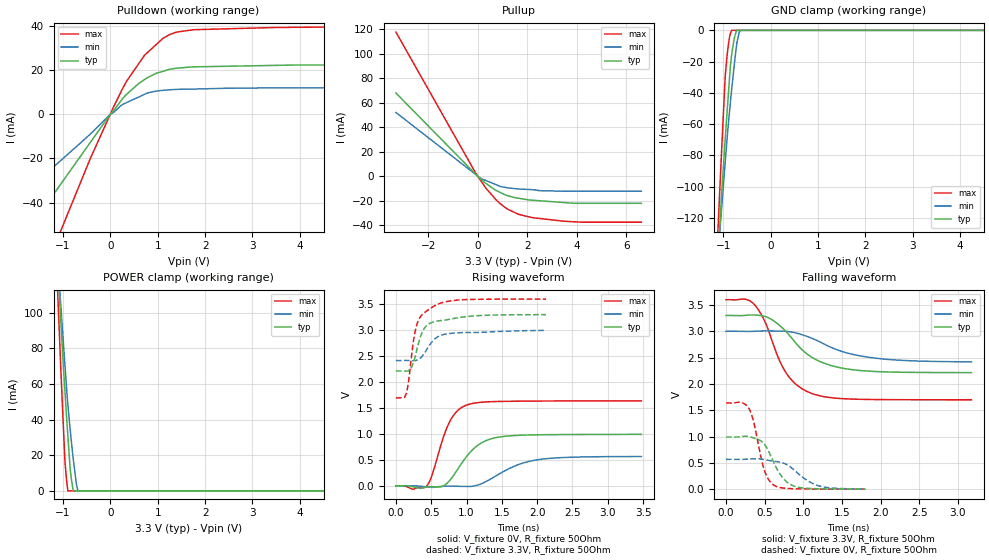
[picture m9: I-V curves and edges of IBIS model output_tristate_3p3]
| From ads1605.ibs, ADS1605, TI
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|   OUTPUT 3.3V Model
[Model]   output_tristate_3p3
Model_type   3-state
Polarity   Non-Inverting
Enable   Active-Low
Vmeas = 1.65
Vref = 1.65
Cref = 15pF
Rref = 50
|   typ   min   max
|   (nom PVT)   (Fast PVT)   (Slow PVT)
|Average
C_comp   2.296e-12   2.043e-12   2.570e-12
|ON state : BUFFER OUTPUT TURNED HIGH
|C_comp   2.372e-12   2.654e-12   2.116e-12
|OFF state: BUFFER in HIGH IMPEDANCE for IOs and 3-state
|C_comp   2.221e-12   2.485e-12   1.971e-12
|Where nom PVT is NOM Process, 3.3V,39C
|   Fast PVT is Strong Process, 3.6V, -40C
|   Slow PVT is Weak Process, 3.0V, 99C
[Voltage Range]   3.3   3   3.6
|Ambient Temperature   25   85   -40
|Junction Temperature
[Temperature Range]   39   99   -40
[Pullup Reference]   3.3   3   3.6
[Pulldown Reference]   0   0   0
[Power Clamp Reference]   3.3   3   3.6
[GND Clamp Reference]   0   0   0
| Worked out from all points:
|   slope of the pulldown table from 0 to 0.495 V, typ, clamps not added: 41.7 ohm
|   slope of the pullup table from 0 to 0.495 V, typ, clamps not added: 60.5 ohm
|   GND clamp passes 1 mA (typ) near -0.73 V on its own axis
|   POWER clamp passes 1 mA (typ) near -0.79 V on its own axis
|   falling waveform, V_fixture 3.3V, R_fixture 50Ohm: 20-80 % time 491ps typ, 647ps min, 355ps max; typ from 3.3 V to 2.21 V
|   rising waveform, V_fixture 0V, R_fixture 50Ohm: 20-80 % time 357ps typ, 516ps min, 253ps max; typ from 0 V to 0.991 V
|   rising waveform, V_fixture 3.3V, R_fixture 50Ohm: 20-80 % time 171ps typ, 211ps min, 144ps max; typ from 2.21 V to 3.3 V
|   falling waveform, V_fixture 0V, R_fixture 50Ohm: 20-80 % time 220ps typ, 309ps min, 152ps max; typ from 0.992 V to 0.002 V
[Pulldown]
|   Voltage   I(typ)   I(min)   I(max)
-3.3V     -99.75mA   -64.03mA   -170.9mA
-429mV    -12.97mA   -9.156mA   -20.36mA
0V        0A         0A         0A
346.8mV   9.051mA    5.259mA    15.01mA
721.2mV   15.6mA     8.938mA    26.62mA
957mV     18.37mA    10.36mA    31.26mA
1.11V     19.37mA    10.77mA    34.28mA
1.254V    20.3mA     11.01mA    35.99mA
1.434V    20.81mA    11.22mA    37.22mA
1.769V    21.38mA    11.33mA    38.18mA
3.45V     22.03mA    11.88mA    39.16mA
6.6V      22.2mA     11.88mA    39.35mA
[GND Clamp]
|   Voltage   I(typ)   I(min)   I(max)
-3.3V     -1.369A    -1.09A     -1.846A
-1.154V   -167.2mA   -161.9mA   -157.2mA
-1.086V   -131.4mA   -134.2mA   -110.6mA
-1.065V   -120.5mA   -125.8mA   -96.82mA
-956.4mV  -68.89mA   -83.51mA   -28.89mA
-877.2mV  -34.64mA   -55.08mA   -6.148mA
-848.1mV  -22.38mA   -45.89mA   -1.939mA
-819.6mV  -15.04mA   -37.07mA   0A
-765.6mV  -4.996mA   -21.71mA   0A
-714mV    -202uA     -8.333mA   0A
-643.5mV  0A         0A         0A
6.6V      0A         0A         0A
[Pullup]
|   Voltage   I(typ)   I(min)   I(max)
-3.3V     67.86mA    51.99mA    117.6mA
0V        0A         0A         0A
332.4mV   -5.843mA   -3.458mA   -9.787mA
764.4mV   -11.7mA    -7.032mA   -19.71mA
1.096V    -15.02mA   -8.994mA   -25.29mA
1.646V    -17.89mA   -10.35mA   -30.99mA
2.194V    -19.48mA   -10.9mA    -33.7mA
2.433V    -19.84mA   -11.69mA   -34.24mA
3.45V     -21.37mA   -12.17mA   -36.56mA
4.202V    -22.03mA   -12.17mA   -37.42mA
6.6V      -22.03mA   -12.17mA   -37.42mA
[POWER Clamp]
|   Voltage   I(typ)   I(min)   I(max)
-3.3V     1.36A      1.083A     1.829A
-1.108V   126.4mA    128.4mA    108.2mA
-1.074V   109mA      114.9mA    86.5mA
-1.057V   100.3mA    108.3mA    75.67mA
-960mV    56.44mA    70.91mA    17.25mA
-927.6mV  42.84mA    58.87mA    6.811mA
-895.2mV  30.19mA    47.86mA    0A
-848.1mV  12.16mA    34.22mA    0A
-792mV    1.441mA    19.79mA    0A
-723mV    0A         5.009mA    0A
-683.1mV  0A         0A         0A
6.6V      0A         0A         0A
[Ramp]
R_load = 50
|   typ   min   max
dV/dt_r   0.595049/3.57434e-10   0.33957/5.17871e-10   0.98264/2.52776e-10
dV/dt_f   0.651402/4.91663e-10   0.35026/6.5499e-10   1.14108/3.55132e-10
[Falling Waveform]
V_fixture = 3.3V
V_fixture_min = 3V
V_fixture_max = 3.6V
R_fixture = 50Ohm
|   Time   V(typ)   V(min)   V(max)
0s        3.3V       3V         3.6V
250ps     3.302V     2.999V     3.609V
375ps     3.308V     3.001V     3.494V
500ps     3.284V     3.007V     3.192V
675ps     3.133V     3.004V     2.501V
775ps     2.997V     2.999V     2.214V
1.075ns   2.54V      2.887V     1.839V
1.4ns     2.333V     2.669V     1.732V
1.825ns   2.245V     2.511V     1.706V
3.175ns   2.215V     2.419V     1.698V
[Rising Waveform]
V_fixture = 0V
V_fixture_min = 0V
V_fixture_max = 0V
R_fixture = 50Ohm
|   Time   V(typ)   V(min)   V(max)
0s        684.4pV    990.5pV    535.6pV
425ps     -21.44mV   -19.32mV   -20.85mV
500ps     -16.42mV   -28.93mV   163.3mV
750ps     85.39mV    -6.353mV   1.204V
875ps     318.3mV    -9.392mV   1.452V
1ns       563.6mV    -12.59mV   1.556V
1.225ns   838mV      49.1mV     1.612V
1.5ns     946.9mV    257.9mV    1.627V
2.1ns     984.6mV    518.7mV    1.634V
3.475ns   991.2mV    564.8mV    1.638V
[Rising Waveform]
V_fixture = 3.3V
V_fixture_min = 3V
V_fixture_max = 3.6V
R_fixture = 50Ohm
|   Time   V(typ)   V(min)   V(max)
0s        2.214V     2.416V     1.698V
150ps     2.21V      2.416V     1.788V
175ps     2.215V     2.415V     1.968V
225ps     2.292V     2.412V     2.553V
250ps     2.381V     2.412V     2.812V
300ps     2.645V     2.424V     3.126V
400ps     3.032V     2.55V      3.332V
500ps     3.143V     2.757V     3.431V
750ps     3.208V     2.935V     3.559V
2.125ns   3.299V     2.996V     3.6V
[Falling Waveform]
V_fixture = 0V
V_fixture_min = 0V
V_fixture_max = 0V
R_fixture = 50Ohm
|   Time   V(typ)   V(min)   V(max)
0s        992.3mV    567.3mV    1.638V
200ps     1V         566.8mV    1.647V
300ps     999.2mV    572.6mV    1.526V
350ps     976.7mV    576.8mV    1.321V
500ps     847.8mV    561.5mV    342.9mV
625ps     485mV      530.2mV    71.15mV
750ps     189.3mV    491.4mV    20.9mV
900ps     50.37mV    339.7mV    8.582mV
1.225ns   8.667mV    54.77mV    3.264mV
1.8ns     2.449mV    5.602mV    1.337mV
